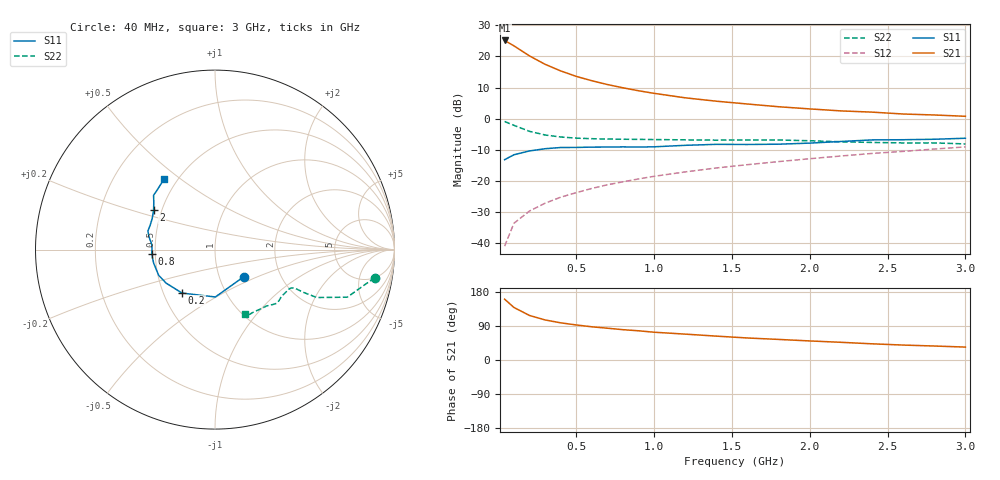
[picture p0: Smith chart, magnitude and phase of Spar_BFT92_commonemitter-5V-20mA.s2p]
! Filename:  BFT92E.S2P  Version:  2.0
! NXP part #: BFT92  Date: May 1990
! Bias condition: Vce=-5V, Ic=-20mA
#  MHz  S  MA  R  50
! Freq  S11  S21  S12  S22  !GUM [dB]
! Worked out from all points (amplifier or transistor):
!   21 points, 40 MHz to 3 GHz, reference 50 ohm
!   highest |S21| = 25.1 dB at 40 MHz (marker M1)
!   |S21| within 3 dB of that: start of sweep to 139.2 MHz
!   unconditionally stable (mu >= 1): 397.9 MHz to 2.137 GHz
!   at 300 MHz: K = 0.94, MSG = 22.3 dB, |S12| = -27.1 dB
!   at 1 GHz: K = 1.12, MAG = 11.2 dB, |S12| = -18.5 dB
!   at 3 GHz: K = 0.89, MSG = 4.9 dB, |S12| = -9.0 dB
!   S11 on the Smith chart (normalised r, x): 40 MHz: 1.30, -0.42; 200 MHz: 0.62, -0.33; 800 MHz: 0.48, -0.02; 2 GHz: 0.45, +0.24; 3 GHz: 0.42, +0.44
40  0.22 -43.8  18.04 160.5  0.009 79.5  0.903 -10.0
100  0.264 -89.6  14.78 138.6  0.021 72.1  0.783 -19.8
200  0.304 -127.2  10.19 117.5  0.033 68.7  0.627 -25.2
300  0.33 -145.5  7.467 105.7  0.044 69.4  0.548 -25.8
400  0.345 -155.5  5.856 98.1  0.055 70.9  0.509 -25.8
500  0.346 -162.2  4.782 92.5  0.065 72.0  0.488 -26.0
600  0.35 -167.5  4.074 87.6  0.076 72.9  0.478 -26.5
700  0.351 -171.8  3.538 83.9  0.087 73.5  0.472 -27.2
800  0.353 -176.3  3.137 80.0  0.097 74.1  0.468 -27.7
900  0.351 179.2  2.812 77.1  0.108 74.2  0.466 -28.9
1000  0.354 175.2  2.554 73.3  0.119 74.2  0.463 -29.8
1200  0.374 169.2  2.165 68.3  0.14 74.4  0.458 -32.3
1400  0.388 164.6  1.911 63.0  0.162 74.2  0.453 -35.3
1600  0.386 159.7  1.722 58.1  0.183 73.7  0.456 -38.5
1800  0.39 153.8  1.557 54.3  0.205 73.6  0.455 -41.2
2000  0.406 147.4  1.437 50.3  0.228 73.0  0.443 -43.8
2200  0.431 142.3  1.335 46.7  0.252 72.6  0.426 -47.5
2400  0.457 138.5  1.276 42.7  0.277 71.4  0.416 -53.0
2600  0.46 135.8  1.19 39.4  0.299 70.4  0.409 -58.0
2800  0.468 131.6  1.148 36.9  0.326 69.7  0.409 -62.0
3000  0.486 125.5  1.094 34.1  0.353 68.0  0.394 -65.3
